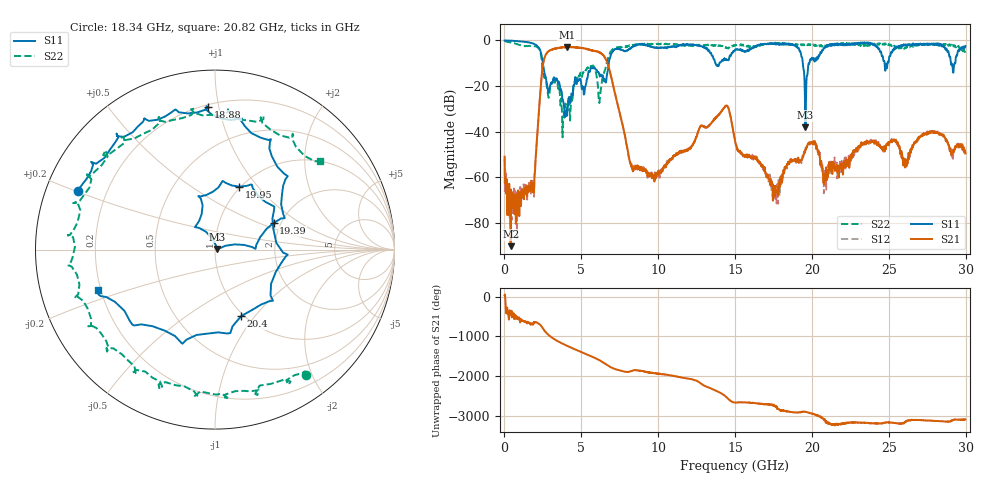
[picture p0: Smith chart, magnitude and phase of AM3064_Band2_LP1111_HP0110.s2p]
# Hz S DB R 50.0
!freq dBS11 angS11 dBS21 angS21 dBS12 angS12 dBS22 angS22
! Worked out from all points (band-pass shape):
!   1600 points, 10 MHz to 29.98 GHz, reference 50 ohm
!   highest |S21| = -2.85 dB at 4.059 GHz (marker M1); lowest = -90.3 dB at 403.6 MHz (marker M2)
!   |S21| within 3 dB of the highest: 2.732 GHz to 6.315 GHz (3.583 GHz wide, 79.2 % of centre)
!   lowest |S11| = -38.1 dB at 19.58 GHz (marker M3), VSWR 1.03, Z = 51.2 + j0.383 ohm
!   |S11| at or under -10 dB: 2.492 GHz to 6.787 GHz (4.295 GHz wide, 92.6 % of centre); 13.72 GHz to 13.97 GHz (256.3 MHz wide, 1.85 % of centre); 19.41 GHz to 19.83 GHz (426.5 MHz wide, 2.17 % of centre)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
!   |S22| runs from -42.5 to -0.1 dB; largest |S21 - S12| = 0.02
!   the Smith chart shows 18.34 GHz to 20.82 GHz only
!   S11 on the Smith chart (normalised r, x): 18.34 GHz: 0.10, +0.20; 18.88 GHz: 0.21, +0.93; 19.39 GHz: 1.83, +0.62; 19.95 GHz: 0.99, +0.81; 20.4 GHz: 0.97, -0.85; 20.82 GHz: 0.19, -0.16
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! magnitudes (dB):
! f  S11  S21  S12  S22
! 10 MHz  0.0  -51.0  -51.8  -0.1
! 403.6 MHz  -0.2  -90.3  -81.0  -0.9
! 1.828 GHz  -1.3  -63.4  -61.8  -2.5
! 2.653 GHz  -15.3  -6.8  -6.7  -16.3
! 4.059 GHz  -31.5  -2.9  -2.8  -31.0
! 5.015 GHz  -20.3  -3.3  -3.3  -15.8
! 6.627 GHz  -17.4  -8.7  -8.7  -10.3
! 8.295 GHz  -3.0  -55.5  -55.0  -2.1
! 10 GHz  -3.3  -57.3  -57.3  -1.6
! 14.37 GHz  -8.6  -28.7  -28.7  -3.2
! 15 GHz  -4.1  -44.3  -44.1  -2.1
! 17.57 GHz  -1.3  -68.6  -66.2  -1.4
! 18.34 GHz  -1.6  -55.6  -55.7  -1.3
! 18.88 GHz  -2.0  -52.4  -52.9  -2.1
! 19.39 GHz  -8.9  -51.6  -50.6  -1.8
! 19.58 GHz  -38.1  -48.4  -48.0  -2.0
! 19.95 GHz  -8.5  -44.9  -44.6  -2.1
! 19.99 GHz  -7.7  -44.5  -44.8  -1.7
! 20.4 GHz  -8.0  -48.4  -49.9  -2.5
! 20.82 GHz  -3.3  -61.1  -57.2  -2.3
! 25 GHz  -9.0  -45.9  -45.8  -1.6
! 29.98 GHz  -2.5  -49.4  -50.1  -4.3
